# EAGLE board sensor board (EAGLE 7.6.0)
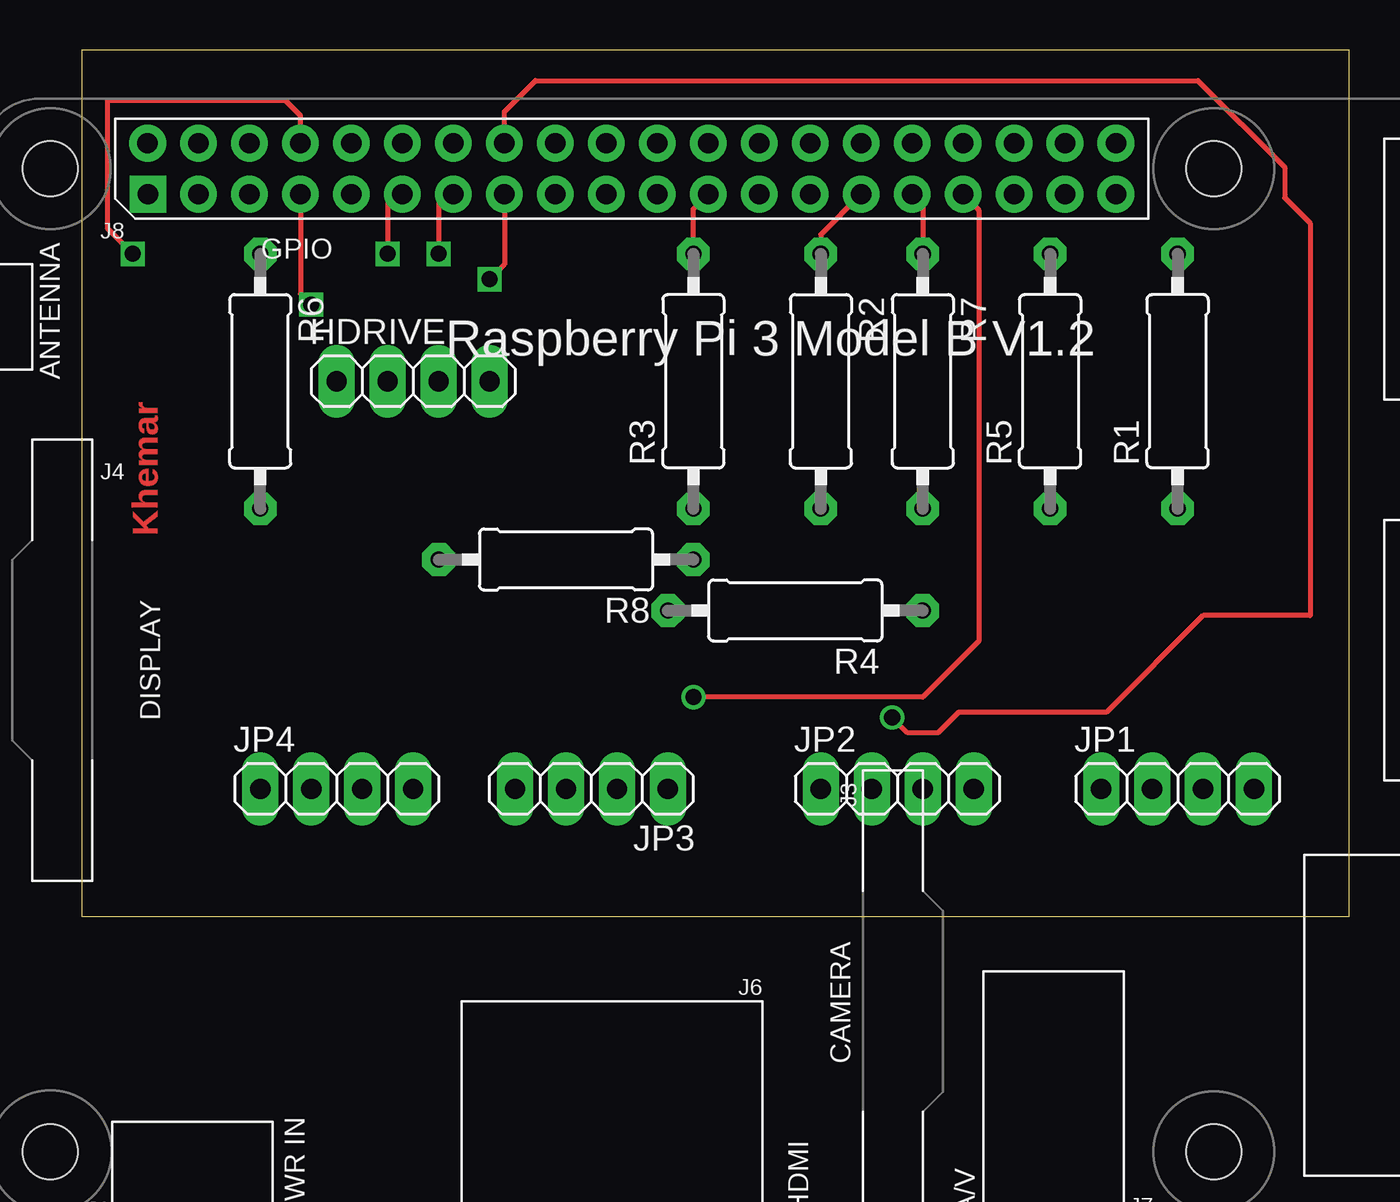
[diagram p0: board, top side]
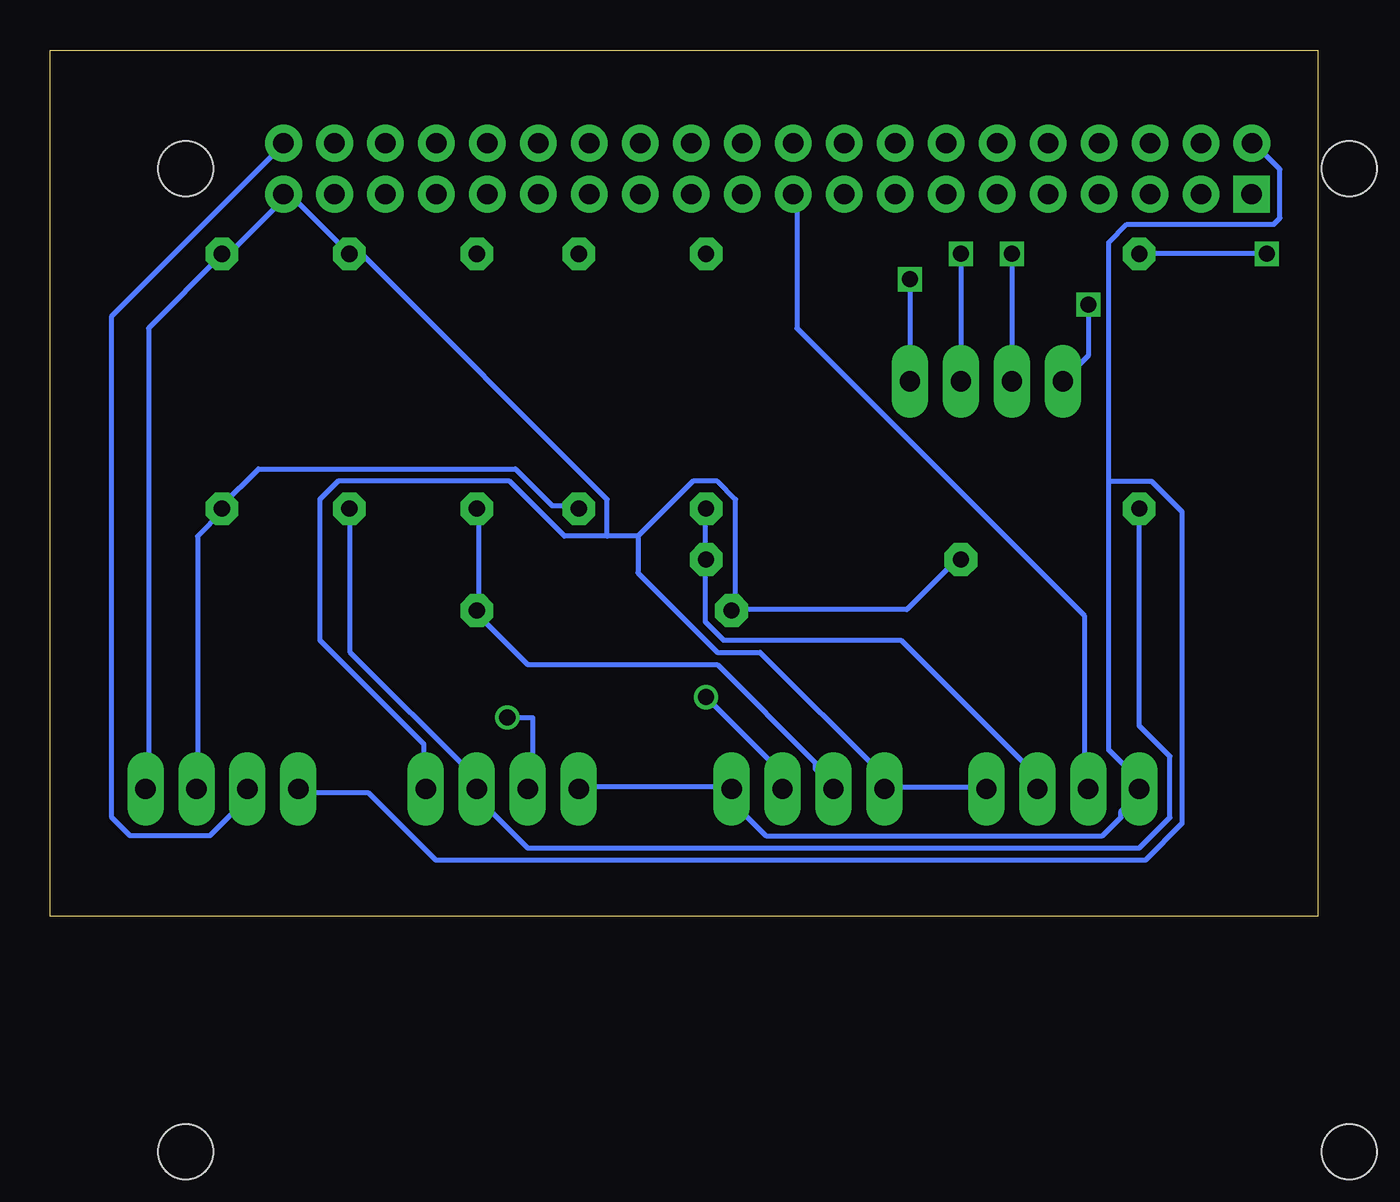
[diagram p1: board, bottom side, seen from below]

Size 63.17 x 43.17 mm. Coordinates in mm from the lower left corner, seen from the top.
Outline: 0,0 63.17,0 63.17,43.17 0,43.17 0,0
Copper layers (1*16): Top 0.035mm / dielectric 1.5mm / Bottom 0.035mm
Design rules "default *": minimum track width 10mil, minimum drill 24mil, track to track 14mil, track to pad 14mil, pad to pad 8mil, via to via 8mil, smd to smd 8mil, copper to edge 40mil, drill to drill 8mil, minimum pad ring 16mil, minimum via ring 8mil, stop-mask expansion 4mil, vias tented up to drill 0mil, thermal gap 10mil

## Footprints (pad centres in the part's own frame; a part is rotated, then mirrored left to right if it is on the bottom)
1X04 = drill 1.016 long: 1 -3.81,0; 2 -1.27,0; 3 1.27,0; 4 3.81,0
RPI3 = drill 1.016 square: P$1 8.37,51.23 | drill 1.016: P$2 8.357,53.772; P$3 10.897,51.232; P$4 10.897,53.772; P$5 13.437,51.232; P$6 13.437,53.772; P$7 15.977,51.232; P$8 15.977,53.772; P$9 18.517,51.232; P$10 18.517,53.772; P$11 21.057,51.232; P$12 21.057,53.772; P$13 23.597,51.232; P$14 23.597,53.772; P$15 26.137,51.232; P$16 26.137,53.772; P$17 28.677,51.232; P$18 28.677,53.772; P$19 31.217,51.232; P$20 31.217,53.772; P$21 33.757,51.232; P$22 33.757,53.772; P$23 36.297,51.232; P$24 36.297,53.772; P$25 38.837,51.232; P$26 38.837,53.772; P$27 41.377,51.232; P$28 41.377,53.772; P$29 43.917,51.232; P$30 43.917,53.772; P$31 46.457,51.232; P$32 46.457,53.772; P$33 48.997,51.232; P$34 48.997,53.772; P$35 51.537,51.232; P$36 51.537,53.772; P$37 54.077,51.232; P$38 54.077,53.772; P$39 56.617,51.232; P$40 56.617,53.772 | hole 2.75: 3.5,3.5; 61.5,3.5; 3.5,52.5; 61.5,52.5
0309/12 = drill 0.813 octagon: 1 -6.35,0; 2 6.35,0

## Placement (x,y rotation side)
HDRIVE  [1X04]  16.51,26.67 0 top
JP1  [1X04]  54.61,6.35 0 top
JP2  [1X04]  40.64,6.35 0 top
JP3  [1X04]  25.4,6.35 180 top
JP4  [1X04]  12.7,6.35 0 top
PCB1  RPI3  [RPI3]  -5.08,-15.24 0 top
R1  1k  [0309/12]  54.61,26.67 90 top
R2  680  [0309/12]  36.83,26.67 270 top
R3  680  [0309/12]  30.48,26.67 90 top
R4  1k  [0309/12]  35.56,15.24 180 top
R5  1k  [0309/12]  48.26,26.67 90 top
R6  680  [0309/12]  8.89,26.67 270 top
R7  680  [0309/12]  41.91,26.67 270 top
R8  1k  [0309/12]  24.13,17.78 180 top

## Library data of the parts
HDRIVE JP1-JP4 = pinhead
PCB1 = e14_Rpi3_RevA
R1-R8 = resistor

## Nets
N$1: JP1.1 JP2.1 JP3.1 JP4.1 PCB1.P$2
N$2: JP4.2 PCB1.P$19
N$3: PCB1.P$23 R3.2
N$4: JP1.3 R1.1 R2.2
N$5: JP1.2 PCB1.P$40
N$6: JP1.4 JP2.4 JP3.4 JP4.4 PCB1.P$39 R1.2 R4.2 R5.2 R8.2
N$7: JP4.3 R3.1 R8.1
N$8: PCB1.P$29 R2.1
N$9: JP2.2 PCB1.P$16
N$10: JP2.3 R5.1 R6.2
N$11: PCB1.P$8 R6.1
N$12: HDRIVE.1 PCB1.P$7
N$13: JP3.3 R4.1 R7.2
N$14: PCB1.P$31 R7.1
N$15: JP3.2 PCB1.P$33
N$16: HDRIVE.2 PCB1.P$11
N$17: HDRIVE.3 PCB1.P$13
N$18: HDRIVE.4 PCB1.P$15

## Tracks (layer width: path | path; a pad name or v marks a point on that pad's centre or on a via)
N$1
  Bottom 0.254: JP2.1 36.63,6.45 29.31,6.45 JP3.1 29.01,6.15 29.01,5.54 27.48,4.01 10.72,4.01 9.8,4.93 9.8,5.23 8.89,6.15 JP4.1 8.89,6.76 10.41,8.28 10.41,21.69 | 10.41,21.69 10.41,33.58 9.5,34.49 2.18,34.49 1.88,34.8 1.88,37.24 3.1,38.46 PCB1.P$2 | 10.41,21.69 8.28,21.69 6.76,20.17 6.76,4.62 8.58,2.79 43.94,2.79 47.3,6.15 50.65,6.15 JP1.1
N$2
  Bottom 0.254: JP4.2 11.63,6.45 11.63,14.99 25.96,29.31 25.96,35.71 PCB1.P$19
N$3
  Top 0.254: R3.2 30.48,35.26 PCB1.P$23
N$4
  Bottom 0.254: R2.2 36.93,20.47 38.15,20.47 39.98,22.3 52.78,22.3 54.61,20.47 R1.1 54.61,20.17 55.83,18.95 55.83,6.45 JP1.3
N$5
  Bottom 0.254: PCB1.P$40 51.56,38.46 60.1,29.92 60.1,4.93 59.18,4.01 55.22,4.01 53.09,6.15 JP1.2
N$6
  Bottom 0.254: JP1.4 58.27,6.45 58.27,29.31 54.61,32.97 R1.2 54.61,33.27 54,33.27 51.56,35.71 PCB1.P$39 51.26,36.02 R5.2 48.21,32.97 47.6,32.97 35.41,20.78 35.41,18.95 | JP4.4 16.51,6.45 21.39,6.45 JP3.4 21.69,6.45 21.69,7.06 27.79,13.16 29.92,13.16 33.88,17.12 33.88,18.95 | 29.01,15.29 20.47,15.29 18.03,17.73 R8.2 | 33.88,18.95 35.41,18.95 | 35.41,18.95 37.54,18.95 40.28,21.69 48.82,21.69 49.73,20.78 49.73,13.77 44.55,8.59 44.55,6.45 JP2.4 | 33.88,18.95 31.14,21.69 29.92,21.69 29.01,20.78 29.01,15.29 | 29.01,15.29 R4.2
N$7
  Bottom 0.254: R3.1 30.53,20.17 30.53,18.03 R8.1 30.53,17.73 30.53,14.68 29.62,13.77 20.78,13.77 14.07,7.06 14.07,6.45 JP4.3
N$8
  Top 0.254: R2.1 36.83,33.98 PCB1.P$29
N$9  (via drill 0.8)
  Top 0.254: PCB1.P$16 21.06,40.11 22.61,41.66 55.63,41.66 59.94,37.34 59.94,35.81 61.21,34.54 61.21,14.99 55.88,14.99 51.05,10.16 43.69,10.16 42.67,9.14 41.15,9.14 v40.39,9.91
  Bottom 0.254: v40.39,9.91 39.12,9.91 39.12,6.6 JP2.2
N$10
  Bottom 0.254: R6.2 8.89,9.5 7.37,7.98 7.37,4.93 8.89,3.4 39.37,3.4 42.11,6.15 JP2.3 42.11,6.45 42.11,7.06 48.21,13.16 48.21,20.17 R5.1
N$11  (via drill 0.8)
  Top 0.254: PCB1.P$8 10.9,39.9 10.16,40.64 1.27,40.64 1.27,34.29 v2.54,33.02
  Bottom 0.254: v2.54,33.02 R6.1
N$12  (via drill 0.8)
  Top 0.254: PCB1.P$7 10.9,31.01 v11.43,30.48
  Bottom 0.254: v11.43,30.48 11.43,27.94 HDRIVE.1
N$13
  Bottom 0.254: R7.2 41.81,20.17 41.81,15.29 R4.1 41.81,14.99 39.37,12.55 29.92,12.55 25.04,7.67 25.04,7.37 24.13,6.45 JP3.3
N$14
  Top 0.254: R7.1 41.91,35.46 PCB1.P$31
  Bottom 0.254: 41.81,33.27 R7.1
N$15  (via drill 0.8)
  Top 0.254: PCB1.P$33 44.7,35.2 44.7,13.72 41.91,10.92 v30.48,10.92
  Bottom 0.254: v30.48,10.92 26.67,7.11 JP3.2
N$16  (via drill 0.8)
  Top 0.254: PCB1.P$11 15.24,35.56 v15.24,33.02
  Bottom 0.254: v15.24,33.02 HDRIVE.2
N$17  (via drill 0.8)
  Top 0.254: PCB1.P$13 17.78,35.56 v17.78,33.02
  Bottom 0.254: v17.78,33.02 HDRIVE.3
N$18  (via drill 0.8)
  Top 0.254: PCB1.P$15 21.06,32.49 v20.32,31.75
  Bottom 0.254: v20.32,31.75 HDRIVE.4

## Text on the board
Top: Khemar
